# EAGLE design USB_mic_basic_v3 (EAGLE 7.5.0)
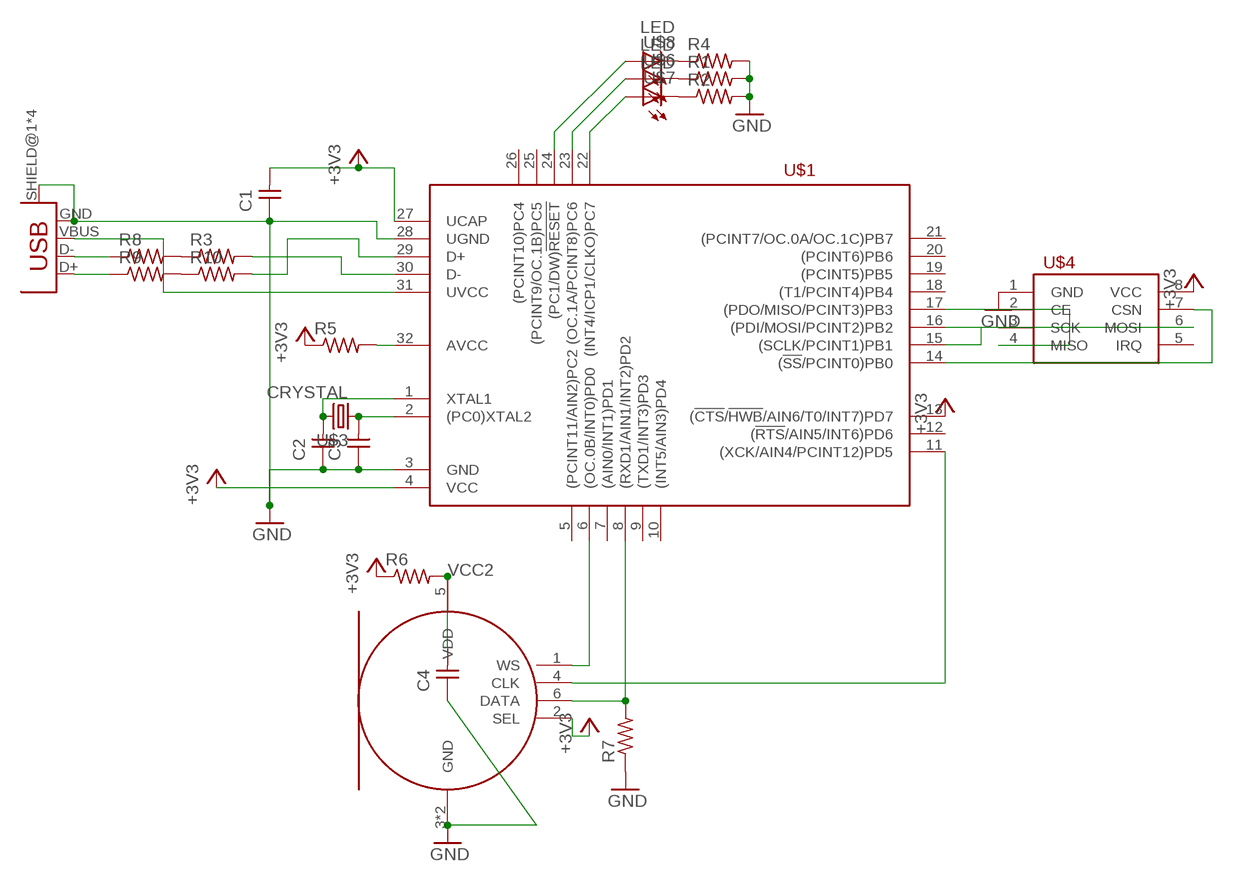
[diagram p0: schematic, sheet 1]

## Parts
C1  CAP-UNPOLARIZEDFAB  [C1206FAB]
C2  CAP-UNPOLARIZEDFAB  [C1206FAB]
C3  CAP-UNPOLARIZEDFAB  [C1206FAB]
C4  CAP-UNPOLARIZEDFAB  [C1206FAB]
R1  RES-US1206FAB  [R1206FAB]
R2  RES-US1206FAB  [R1206FAB]
R3  RES-US1206FAB  [R1206FAB]
R4  RES-US1206FAB  [R1206FAB]
R5  RES-US1206FAB  [R1206FAB]
R6  RES-US1206FAB  [R1206FAB]
R7  RES-US1206FAB  [R1206FAB]
R8  RES-US1206FAB  [R1206FAB]
R9  RES-US1206FAB  [R1206FAB]
R10  RES-US1206FAB  [R1206FAB]
U$1  ATMEGA16U2-TQ  [TQFP32-08THIN]
U$2  USB_MINIB  [USB_MINIB]
U$3  CRYSTAL  [2-SMD-5X3MM]
U$4  NRF24L01+  [2X04_THRU]
U$5  MEMS_MIC_SPH0645LM4H-BI2S  [MIC_BOTTOM_PORT]
U$6  LED  [LED1206]
U$7  LED  [LED1206]
U$8  LED  [LED1206]

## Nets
+3V3: C1.2 R5.1 R6.1 U$1.4(VCC) U$1.13((!CTS!/!HWB!/AIN6/T0/INT7)PD7) U$1.27(UCAP) U$4.8(VCC) U$5.2(SEL)
GND: C1.1 C2.1 C3.1 C4.1 R1.2 R2.2 R4.2 R7.1 U$1.3(GND) U$1.28(UGND) U$2.GND U$2.SHIELD@1(SHIELD) U$2.SHIELD@2(SHIELD) U$2.SHIELD@3(SHIELD) U$2.SHIELD@4(SHIELD) U$4.1(GND) U$5.3(GND) U$5.P$1(GND)
N$1: R3.2 U$1.30(D-)
N$2: R10.2 U$1.29(D+)
N$3: U$1.31(UVCC) U$2.VBUS
N$4: U$1.22((INT4/ICP1/CLKO)PC7) U$7.1(A)
N$5: U$1.23((OC.1A/PCINT8)PC6) U$6.1(A)
N$6: C2.2 U$1.1(XTAL1) U$3.P$2
N$7: C3.2 U$1.2((PC0)XTAL2) U$3.P$1
N$8: R1.1 U$6.2(C)
N$9: U$1.15((SCLK/PCINT1)PB1) U$4.3(SCK)
N$10: U$1.17((PDO/MISO/PCINT3)PB3) U$4.4(MISO)
N$11: U$1.16((PDI/MOSI/PCINT2)PB2) U$4.6(MOSI)
N$12: U$1.14((!SS!/PCINT0)PB0) U$4.7(CSN)
N$13: U$1.11((XCK/AIN4/PCINT12)PD5) U$5.4(CLK)
N$14: R7.2 U$1.8((RXD1/AIN1/INT2)PD2) U$5.6(DATA)
N$15: R2.1 U$7.2(C)
N$16: U$1.6((OC.0B/INT0)PD0) U$5.1(WS)
N$17: R8.1 U$2.D-
N$18: R4.1 U$8.2(C)
N$19: U$1.24((PC1/DW)!RESET) U$8.1(A)
N$20: R5.2 U$1.32(AVCC)
N$21: R9.1 U$2.D+
N$22: R3.1 R8.2
N$23: R9.2 R10.1
VCC2: C4.2 R6.2 U$5.5(VDD)
Unconnected: U$1.5((PCINT11/AIN2)PC2) U$1.7((AIN0/INT1)PD1) U$1.9((TXD1/INT3)PD3) U$1.10((INT5/AIN3)PD4) U$1.12((!RTS!/AIN5/INT6)PD6) U$1.18((T1/PCINT4)PB4) U$1.19((PCINT5)PB5) U$1.20((PCINT6)PB6) U$1.21((PCINT7/OC.0A/OC.1C)PB7) U$1.25((PCINT9/OC.1B)PC5) U$1.26((PCINT10)PC4) U$4.2(CE) U$4.5(IRQ)

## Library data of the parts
C1-C4 = fab:CAP-UNPOLARIZED
R1-R10 = fab:RES-US: Resistor (US Symbol)
U$1 = fab:ATMEGA16U2
U$2 = fab:USB_MINIB
U$3 = fab:CRYSTAL
U$4 = fab:NRF24L01+: nRF24L01+ 2.4GHz Wireless Transceiver module
U$5 = fab:MEMS_MIC_SPH0645LM4H-B
U$6-U$8 = fab:LED: LED

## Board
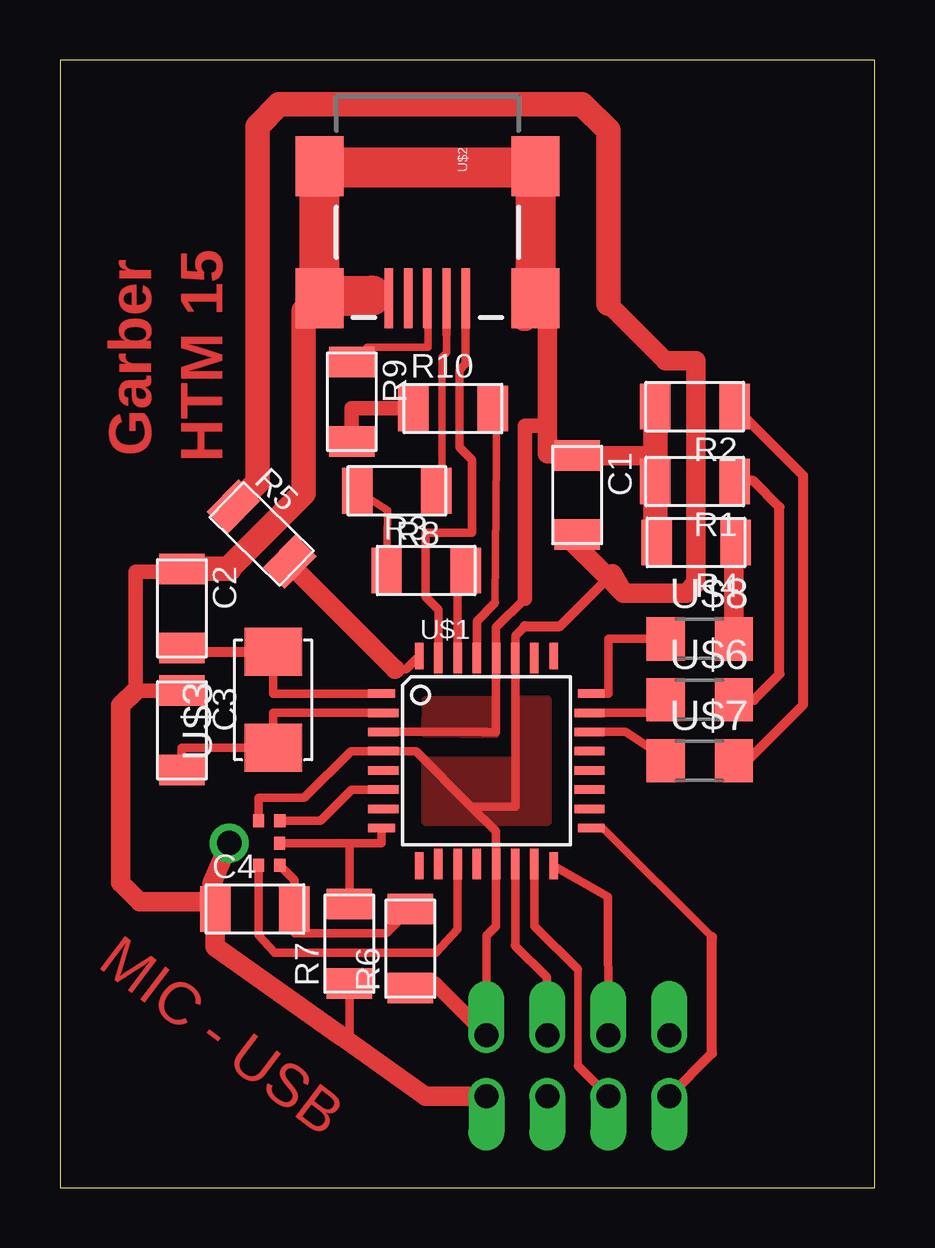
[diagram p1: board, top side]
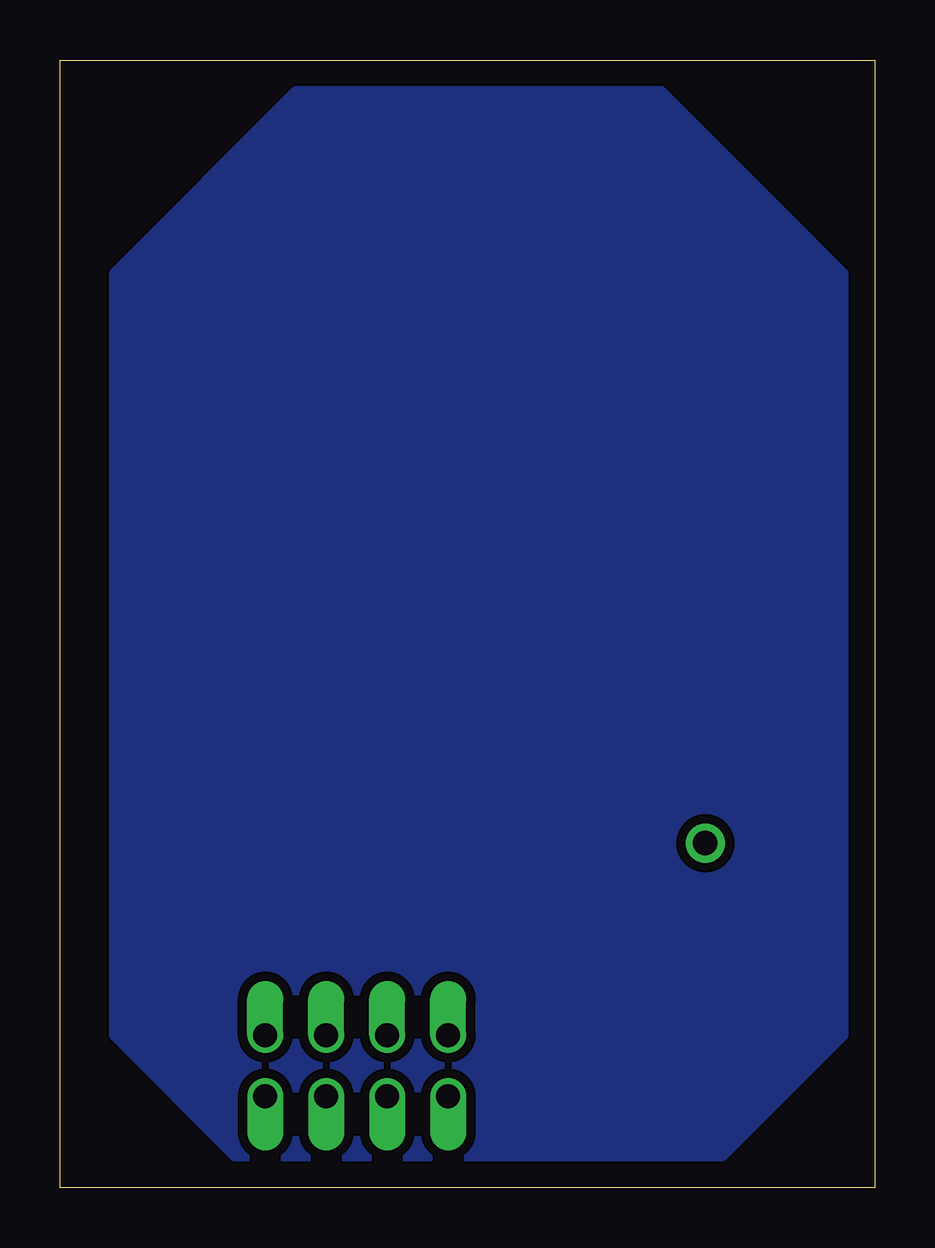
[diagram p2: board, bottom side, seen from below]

Size 33.96 x 46.98 mm. Coordinates in mm from the lower left corner, seen from the top.
Outline: 0,0 33.96,0 33.96,46.98 0,46.98 0,0
Copper layers (1*16): Top 0.035mm / dielectric 1.5mm / Bottom 0.035mm
Design rules "fab": minimum track width 0.3mm, minimum drill 32mil, track to track 0.397mm, track to pad 0.397mm, pad to pad 0.397mm, via to via 0.397mm, smd to smd 0.315mm, copper to edge 40mil, drill to drill 16mil, minimum pad ring 10mil, minimum via ring 8mil, stop-mask expansion 4mil, vias tented up to drill 0mil, thermal gap 10mil

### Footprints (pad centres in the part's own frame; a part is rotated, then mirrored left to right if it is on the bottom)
C1206FAB = smd 1.27 x 1.905: 1 -1.651,0; 2 1.651,0
R1206FAB = smd 1.27 x 1.905: 1 -1.651,0; 2 1.651,0
TQFP32-08THIN = smd 1.118 x 0.356: 1 -4.369,2.8; 8 -4.369,-2.8; 17 4.369,-2.8; 24 4.369,2.8 | smd 1.27 x 0.356: 2 -4.293,2; 3 -4.293,1.2; 4 -4.293,0.4; 5 -4.293,-0.4; 6 -4.293,-1.2; 7 -4.293,-2; 18 4.293,-2; 19 4.293,-1.2; 20 4.293,-0.4; 21 4.293,0.4; 22 4.293,1.2; 23 4.293,2 | smd 0.356 x 1.118: 9 -2.8,-4.369; 16 2.8,-4.369; 25 2.8,4.369; 32 -2.8,4.369 | smd 0.356 x 1.27: 10 -2,-4.293; 14 1.2,-4.293; 15 2,-4.293; 26 2,4.293; 27 1.2,4.293; 31 -2,4.293 | smd 0.35 x 1.27: 11 -1.2,-4.293; 12 -0.4,-4.293; 13 0.4,-4.293; 28 0.4,4.293; 29 -0.4,4.293; 30 -1.2,4.293
USB_MINIB = smd 2.5 x 0.35: D+ 3.77,0; D- 3.77,0.8; GND 3.77,-1.6; ID 3.77,-0.8; VBUS 3.77,1.6 | smd 2.5 x 2: SHIELD@1 -1.73,-4.5; SHIELD@2 -1.73,4.5; SHIELD@3 3.77,4.5; SHIELD@4 3.77,-4.5
2-SMD-5X3MM = smd 2 x 2.4: P$1 -2,0; P$2 2,0
2X04_THRU = drill 1 pad 1.27 offset: 1 -1.27,3.81; 2 -1.27,1.27; 3 -1.27,-1.27; 4 -1.27,-3.81; 5 1.27,-3.81; 6 1.27,-1.27; 7 1.27,1.27; 8 1.27,3.81
MIC_BOTTOM_PORT = smd 0.54 x 0.46: 1 -0.929,2.106; 2 -0.931,1.221; 4 0.931,1.22; 5 0.93,2.105; 6 0,2.102 | smd 1.624 x 1.624: 3 0,0 | drill 1.024 pad 1.624: P$1 0,0
LED1206 = smd 1.6 x 1.803: 1 -1.422,0; 2 1.422,0

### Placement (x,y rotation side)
C1  21.56,28.85 270 top
C2  5.08,24.13 270 top
C3  5.08,19.05 270 top
C4  8.13,11.61 0 top
R1  26.47,29.41 180 top
R2  26.47,32.54 180 top
R3  15.27,25.7 0 top
R4  26.52,26.87 180 top
R5  8.41,27.23 315.6 top
R6  14.61,9.96 90 top
R7  12.06,10.16 90 top
R8  14.05,29.03 180 top
R9  12.17,32.74 270 top
R10  16.38,32.46 0 top
U$1  17.78,17.78 0 top
U$2  15.32,40.82 270 top
U$3  8.89,20.32 90 top
U$4  21.59,5.08 90 top
U$5  7.06,14.35 270 top
U$6  26.67,20.32 0 top
U$7  26.67,17.78 0 top
U$8  26.67,22.86 0 top

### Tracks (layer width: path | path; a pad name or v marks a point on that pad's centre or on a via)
+3V3
  Top 0.356: U$4.8 17.78,10.49 18.18,10.89 U$1.13 18.18,14.84 17.14,15.88 | 17.14,15.88 14.84,18.18 U$1.4 12.13,18.18 10.19,16.23 8.28,16.23 U$5.2 | 17.14,15.88 18.98,15.88 U$1.27 18.98,22.99 19.38,23.39
  Top 0.406: 19.38,23.39 20.85,23.39 22.86,25.4
  Top 0.61: U$4.8 15.62,8.51 R6.1
  Top 0.813: 23.04,25.58 23.5,24.77 | 23.5,24.77 26.11,24.77 26.52,25.17 26.52,34.44 25.25,34.44 22.86,36.83 | C1.2 21.03,27.23 22.86,25.4 23.5,24.77
  Top 1.016: 22.86,36.83 22.86,44.04 21.77,45.14 9.14,45.14 8.23,44.22 8.23,29.39 R5.1
  pour Top: 15.24,17.78 15.24,15.24 20.32,15.24 20.32,20.32 19.05,20.32 19.05,17.78
BACK
  pour Bottom: 31.75,38.1 31.75,6.35 26.67,1.27 6.35,1.27 1.27,6.35 1.27,38.1 8.89,45.72 24.13,45.72
GND
  Top 0.305: U$2.SHIELD@3 19.13,36.36
  Top 0.356: U$2.GND U$2.SHIELD@4 | U$1.3 17.78,18.98 17.63,18.97 18.18,18.97 U$1.28 18.18,23.34 19.38,24.54 | 19.13,36.36 19.46,35.99 | U$2.SHIELD@2 19.82,42.49 19.13,42.49 | 10.9,42.49 10.9,42.55 U$2.SHIELD@1 | R7.1 12.06,6.29 11.75,6.29
  Top 0.61: C3.1 3.15,20.7 3.15,25.65 5.08,25.65 C2.1 | 19.33,36.09 19.46,35.99 | 19.38,24.54 19.38,31.75 20.32,31.75
  Top 0.813: 3.15,20.7 2.54,20.09 2.54,12.7 3.33,11.91 6.17,11.91 C4.1 | U$5.P$1 6.35,12.7 C4.1 | U$4.1 15.24,3.81 11.75,6.29 6.48,10.03 C4.1 | 19.33,36.09 19.33,36.83 20.32,36.83 20.32,31.75 20.32,30.58 C1.1 21.03,30.48 24.82,30.48
  Top 1.016: C2.1 7.04,25.78 | 7.04,25.78 7.07,25.78 | R2.2 24.82,30.48 R1.2 24.82,26.92 R4.2 | 7.04,25.78 7.04,25.81 10.16,28.93 10.16,36.52 10.74,37.11 10.81,37.05 U$2.SHIELD@4
  Top 1.676: U$2.SHIELD@1 U$2.SHIELD@4 10.93,37.16 13.01,37.16 | U$2.SHIELD@2 U$2.SHIELD@3 | 19.58,42.49 19.13,42.49 10.9,42.49 10.9,42.47
  pour Top: 15.21,18.9 15.24,20.32 18.14,20.32 18.16,18.87
N$1
  Top 0.356: R3.2 16.58,25.57 U$1.30
N$2
  Top 0.305: 18.14,24.36 18.21,32.46 R10.2
  Top 0.356: 18.14,24.36 17.38,23.6 U$1.29
N$3
  Top 0.356: U$2.VBUS 16.92,34.31 16.66,34.06 16.66,30.84 17.17,30.33 17.17,27.28 15.24,27.28 15.24,24.61 15.78,24.07 U$1.31
N$4
  Top 0.356: U$1.22 23.57,18.98 25.4,17.78
  Top 1.016: U$7.1 25.4,17.78
N$5
  Top 0.356: U$6.1 24.71,19.78 U$1.23
N$6
  Top 0.356: U$1.1 8.89,20.58 U$3.P$2
  Top 0.406: C2.2 5.24,22.32 U$3.P$2
N$7
  Top 0.356: U$1.2 8.89,19.78 U$3.P$1 5.08,18.32 C3.2
N$8
  Top 0.406: U$6.2 28.93,20.32 30,21.39 30,28.35 28.91,29.44 28.14,29.44 R1.1
N$9
  Top 0.305: 21.59,5.08 21.59,9.09
  Top 0.356: U$4.3 21.59,5.08 | 21.59,9.09 19.78,10.89 U$1.15
N$10
  Top 0.305: 27.18,10.44 22.64,14.98 U$1.17
  Top 0.406: U$4.4 27.18,5.59 27.18,10.44
N$11
  Top 0.356: U$4.6 22.84,12.12 U$1.16
N$12
  Top 0.356: U$4.7 20.3,8.76 18.97,10.08 18.98,10.23 U$1.14
N$13
  Top 0.356: U$5.4 8.28,10.52 8.94,9.78 15.67,9.78 16.58,10.76 U$1.11
N$14
  Top 0.356: U$5.6 12.06,14.35 | U$1.8 13.41,14.35 12.7,14.35 12.06,14.35 | R7.2 12.06,14.35
N$15
  Top 0.406: U$7.2 28.65,17.78 30.99,20.12 30.99,29.67 R2.1
N$16
  Top 0.356: U$5.1 10.86,15.28 12.16,16.58 U$1.6
N$17
  Top 0.305: 16.12,35.55 16.12,34.78 15.93,34.59 15.93,29.18 15.79,28.45 R8.1
  Top 0.356: U$2.D- 16.12,35.55
N$18
  Top 0.813: U$8.2 28.09,26.87 R4.1
N$19
  Top 0.356: U$8.1 22.86,22.86 22.86,20.58 U$1.24
N$20
  Top 0.356: 13.97,21.59 14.42,21.59 U$1.32
  Top 0.813: R5.2 9.59,25.97 13.97,21.59
N$21
  Top 0.305: U$2.D+ 15.34,35 12.8,35 12.78,34.39 R9.1
N$22
  Top 0.305: R3.1 13.66,28.22 R8.2
N$23
  Top 0.61: R9.2 12.17,32.46 R10.1
VCC2
  Top 0.356: U$5.5 9.78,12.81 C4.2 9.78,10.59 13.59,10.59 R6.2

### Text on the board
Top: Garber | HTM 15 | MIC - USB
